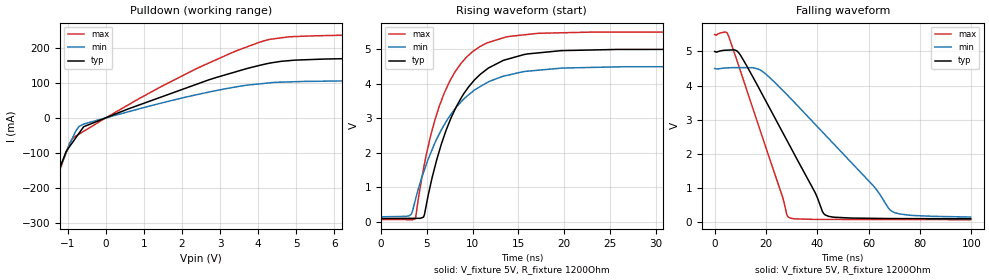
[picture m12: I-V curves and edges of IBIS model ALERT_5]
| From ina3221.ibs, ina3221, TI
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[Model]   ALERT_5
Model_type   Open_drain
Polarity   Non-Inverting
Vmeas = 2.5
Vref = 2.5
Cref = 2pF
Rref = 1200
|   typ   min   max
|   (nom PVT)   (Fast PVT)   (slow PVT)
|   ON state : BUFFER OUTPUT TURNED HIGH
C_comp   1.191E-12   9.774E-13   1.374E-12
|   OFF state: BUFFER OUTPUT TURNED LOW
|C_comp   9.333E-13   8.396E-13   1.009E-12
| Where   nom PVT is  Nominal Process, 3.3V, 25C
|   Fast PVT is Strong Process, 3.6V, -40C
|   Slow PVT is Weak Process, 3.0V, 85C
|C_comp - from L-C Tank method, L = 1nH, peak frequency
[Voltage Range]   5   4.5   5.5
|Ambient Temperature Range   27   85   -40
[Temperature Range]   30   88   -40
[Pullup Reference]   5   4.5   5.5
[Pulldown Reference]   0   0   0
[Power Clamp Reference]   5   4.5   5.5
[GND Clamp Reference]   0   0   0
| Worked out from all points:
|   slope of the pulldown table from 0 to 0.75 V, typ, clamps not added: 23.6 ohm
|   falling waveform, V_fixture 5V, R_fixture 1200Ohm: 20-80 % time 21ns typ, 32.8ns min, 14.5ns max; typ from 5 V to 0.097 V
|   rising waveform, V_fixture 5V, R_fixture 1200Ohm: 20-80 % time 4.51ns typ, 5.19ns min, 3.89ns max; typ from 0.097 V to 5 V
[Pulldown]
|   Voltage   I(typ)   I(min)   I(max)
-5V       -1.382A    -1.301A    -1.544A
-1.82V    -328.7mA   -318.9mA   -347.9mA
-1.043V   -96.09mA   -99.64mA   -99.57mA
-941.1mV  -80.48mA   -73.35mA   -70.57mA
-698.9mV  -43.26mA   -24.35mA   -46.18mA
-583.7mV  -25.55mA   -17.95mA   -38.56mA
579.8mV   25.14mA    17.03mA    36.47mA
2.437V    98.11mA    67.32mA    143.5mA
4.023V    149.5mA    96.92mA    215.6mA
4.977V    165mA      103.3mA    232.4mA
8.654V    173.4mA    108.8mA    242.6mA
9.985V    183.9mA    118.4mA    260.1mA
[Ramp]
R_load = 1200
|   typ   min   max
dV/dt_r   2.94189/4.49917e-009   2.61114/5.17621e-009   3.25746/3.87921e-009
dV/dt_f   2.94188/2.10145e-008   2.61095/3.28253e-008   3.25746/1.44358e-008
[Falling Waveform]
V_fixture = 5V
V_fixture_min = 4.5V
V_fixture_max = 5.5V
R_fixture = 1200Ohm
C_fixture = 0F
|   Time   V(typ)   V(min)   V(max)
0s        5V         4.5V       5.5V
4.178ns   5.036V     4.517V     5.572V
5.32ns    5.04V      4.521V     5.469V
10.07ns   4.887V     4.527V     4.419V
18.21ns   3.787V     4.435V     2.576V
28.79ns   2.303V     3.685V     142mV
43.16ns   205.3mV    2.546V     79.57mV
62.29ns   109.7mV    1.024V     76.64mV
69.22ns   103.7mV    307.5mV    75.57mV
99.73ns   96.87mV    148.4mV    70.9mV
[Rising Waveform]
V_fixture = 5V
V_fixture_min = 4.5V
V_fixture_max = 5.5V
R_fixture = 1200Ohm
C_fixture = 0F
|   Time   V(typ)   V(min)   V(max)
0s        96.84mV    148.1mV    70.89mV
3.089ns   102.7mV    179mV      65.66mV
3.734ns   103.9mV    621.5mV    89.92mV
4.637ns   138.3mV    1.431V     1.535V
6.348ns   2.038V     2.541V     3.339V
8.203ns   3.328V     3.314V     4.39V
10.82ns   4.271V     3.917V     5.08V
13.58ns   4.695V     4.232V     5.35V
25.86ns   4.995V     4.49V      5.496V
99.73ns   5V         4.5V       5.5V
